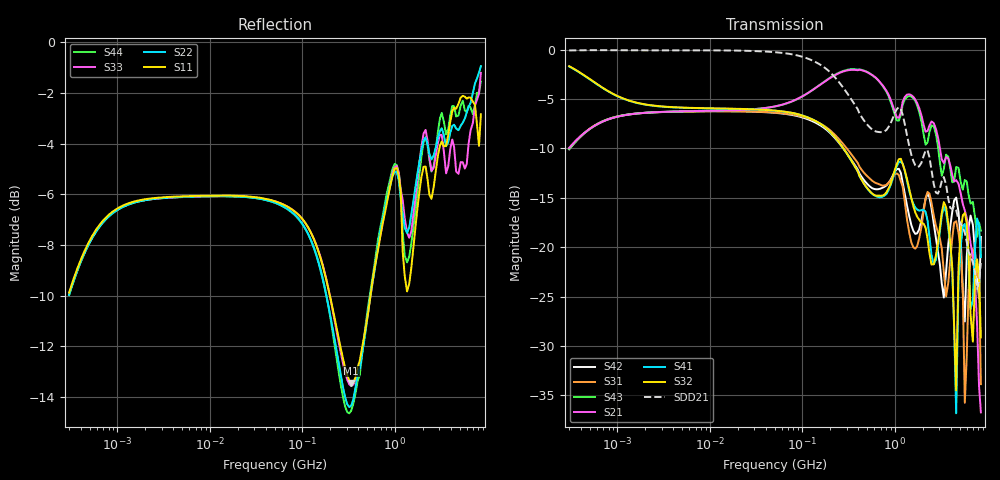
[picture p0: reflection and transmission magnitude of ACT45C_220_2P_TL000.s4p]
! S-Parameter Data Generated by TDK Corporation
! Copyright(C) 2025 TDK Corporation.
! All Rights Reserved.
! TDK P/N: ACT45C-220-2P-TL000 (Signal Line Common Mode Choke/Filter)
! Property: |Zc|=1200ohm at 10MHz
! Size(LxWxT): 4.5x3.2x2.8mm
! Model Type: s2p (Touchstone File Format Version 1.0)
! Frequency: DC=Yes Start=0.3MHz Stop=8500MHz 202points Log-sweep
! Model Generated on July 30, 2025
! Terms and conditions regarding TDK Simulation Models:
! 1)This simulation model is being provided solely for informational
!  purposes. Please refer to the specifications of the products in
!  terms of detailed characteristics of such products.
! 2)In no event shall TDK Corporation of any of its subsidiaries be
!  liable for any loss or damage arising, directly or indirectly,
!  from any information contained in this simulation model, including,
!  but not limited to loss or damages arising from any inaccuracies,
!  omissions or errors in connection with such information.
! 3)Any and all copyrights on this simulation model are owned by
!  TDK Corporation.  Duplication or redistribution of this simulation
!  model without prior written permission from TDK Corporation
!  is prohibited.
! 4)This simulation model is subject to any modification or change
!  without any prior notice.
! 5)Neither TDK Corporation nor any of its subsidiaries shall make any
!  warranty, express or implied, including but not limited to the
!  correctness, implied warranties of merchantability and fitness for
!  a particular purpose with respect to this simulation models.
! 6)The use of this simulation model shall be deemed to have consented
!  to the terms and conditions hereof.
! Port Assignments:
!  1 ---@@@--- 4
!  2 ---@@@--- 3
! Applicable Conditions:
!  Temperature = 25 degC
!  DC Bias Current = 0 A
!  Small Signal Operation
# Hz S MA R 50
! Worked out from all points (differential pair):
!   201 points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, 300 kHz to 8.5 GHz, reference 50 ohm
!   strongest paths, dB at 300 kHz, 3.892 MHz, 50.5 MHz, 655.2 MHz, 8.5 GHz:
!     S32: -1.7, -5.8, -6.2, -14.8, -29.1
!     S41: -1.7, -5.8, -6.2, -14.9, -21.0
!     S21: -10.0, -6.3, -5.7, -3.1, -36.7
!     S43: -10.1, -6.3, -5.8, -3.1, -18.3
!     S31: -10.0, -6.3, -6.4, -13.6, -33.9
!     S42: -10.1, -6.3, -6.4, -14.1, -19.0
!   taken as a pair (ports 2,1 in; 3,4 out), SDD21 dB: -0.1, -0.1, -0.3, -8.3, -21.6
!   lowest |S11| = -13.4 dB at 336.5 MHz (marker M1), VSWR 1.54, Z = 77 - j0.612 ohm
!   |S11| at or under -10 dB: 198.1 MHz to 544.6 MHz (346.4 MHz wide, 93.3 % of centre)
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300000  0.3207 48.4  0.3174 49.6  0.3162 -130.6  0.8267 -16.5
        0.3179 49.8  0.3176 48.5  0.8263 -17.3  0.3168 -129.8
        0.3161 -130.0  0.8247 -16.7  0.318 48.5  0.3167 50.9
        0.8223 -16.6  0.3128 -130.0  0.3144 50.0  0.3171 49.7
3.364691e8  0.2126 -1.0  0.7887 -8.5  0.2942 82.3  0.2732 -98.6
            0.7895 -8.7  0.1918 4.8  0.2729 -99.2  0.2755 77.6
            0.296 82.1  0.2754 -99.2  0.2099 -0.3  0.7953 -8.6
            0.2746 -98.7  0.2776 77.6  0.7964 -8.5  0.1876 5.7
3.970576e9  0.6973 -54.8  0.2587 -100.1  0.08797 69.9  0.09913 -31.5
            0.2588 -99.7  0.6638 -59.4  0.1064 -33.4  0.1248 63.6
            0.08615 69.2  0.1049 -32.2  0.6168 -59.6  0.2541 -83.6
            0.1017 -31.6  0.1277 63.3  0.2484 -84.6  0.7181 -63.7
4.594953e9  0.7396 -67.6  0.2189 -106.7  0.1402 -15.8  0.01422 64.2
            0.2185 -106.6  0.6757 -78.4  0.01721 83.2  0.1685 -10.6
            0.1353 -14.0  0.01883 63.5  0.5558 -82.3  0.2699 -76.2
            0.01442 66.2  0.1782 -10.8  0.255 -78.7  0.7139 -80.6
5.42226e9  0.7839 -82.7  0.1666 -130.4  0.06077 -106.1  0.1166 -12.5
           0.1654 -130.4  0.6944 -102.7  0.1471 -20.9  0.05489 -72.4
           0.05862 -106.4  0.1447 -27.5  0.5795 -104.3  0.2145 -97.3
           0.1275 -13.5  0.0592 -73.8  0.1956 -96.3  0.7666 -100.3
8.115653e9  0.6245 -162.4  0.02042 -41.9  0.07799 -163.8  0.1405 -127.1
            0.01991 -42.7  0.8719 -109.0  0.07488 -90.1  0.05802 -62.3
            0.0693 -171.4  0.07156 -97.9  0.7929 -103.5  0.1186 -118.0
            0.1287 -118.6  0.05507 -53.8  0.1335 -124.7  0.7951 -140.3
8.5e9  0.7211 -171.9  0.01512 -78.5  0.01766 -104.1  0.09093 -136.6
       0.01458 -79.5  0.8972 -98.6  0.03767 -110.6  0.1129 -37.7
       0.02025 -81.0  0.03496 -101.2  0.8704 -91.8  0.1157 -126.4
       0.08905 -127.5  0.1127 -28.4  0.1212 -137.0  0.8363 -137.0
